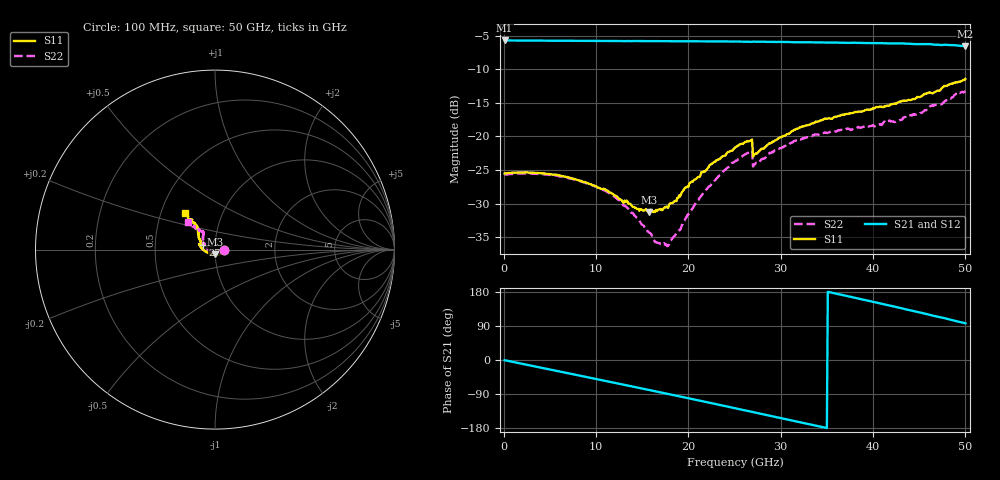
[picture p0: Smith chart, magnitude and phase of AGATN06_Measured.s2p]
! Filename4Jim: AG16_W2_AGATN06_B_0715_LRM_1BW_LRM.s2p
! Calibration: AG02 LRM + TRL
! Notes:
! Row:7, Col:15
! Probes: nan
! Prober: MPI TS150
! Date: 2023-09-21 10:47:37
! DC: None
# GHz S dB R 50
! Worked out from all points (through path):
!   500 points, 100 MHz to 50 GHz, reference 50 ohm
!   highest |S21| = -5.74 dB at 100 MHz (marker M1); lowest = -6.6 dB at 50 GHz (marker M2)
!   group delay of S21, straight-line fit = 14.5 ps
!   lowest |S11| = -31.3 dB at 15.7 GHz (marker M3), VSWR 1.06, Z = 50 - j2.71 ohm
!   |S11| at or under -10 dB: start of sweep to end of sweep
!   |S22| runs from -36.3 to -13.3 dB; largest |S21 - S12| = 0.00059
!   S11 on the Smith chart (normalised r, x): 100 MHz: 1.11, +0.00; 27 GHz: 0.88, +0.04; 50 GHz: 0.66, +0.29
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0.1  -25.54 0.1  -5.74 -0.5  -5.74 -0.5  -25.72 0.2
4.2  -25.52 -5.8  -5.77 -21.1  -5.77 -21.1  -25.64 -3.0
8.5  -26.72 -18.8  -5.79 -42.6  -5.79 -42.6  -26.77 -11.5
12.1  -28.87 -41.1  -5.81 -60.7  -5.81 -60.7  -29.09 -26.6
14.5  -30.82 -68.6  -5.82 -72.8  -5.82 -72.7  -32.23 -45.4
15.7  -31.33 -89.2  -5.82 -78.8  -5.82 -78.8  -34.27 -62.2
16.4  -31.26 -102.9  -5.83 -82.5  -5.83 -82.5  -35.72 -77.4
16.8  -30.90 -110.2  -5.83 -84.6  -5.83 -84.5  -35.90 -87.4
17.9  -30.22 -128.2  -5.85 -90.1  -5.85 -90.1  -36.04 -116.9
22  -24.96 -172.1  -5.88 -111.3  -5.88 -111.3  -27.86 176.0
25.1  -21.61 169.1  -5.89 -127.5  -5.89 -127.4  -23.64 157.5
26.7  -20.64 160.2  -5.93 -135.8  -5.93 -135.8  -22.26 150.8
27  -23.01 159.1  -5.91 -137.5  -5.91 -137.5  -24.49 154.4
27.2  -22.66 157.7  -5.91 -138.6  -5.91 -138.5  -24.16 153.4
29.5  -20.55 149.3  -5.94 -150.6  -5.95 -150.6  -22.03 143.4
33.4  -18.08 137.5  -6.02 -171.2  -6.02 -171.2  -19.97 131.2
37.7  -16.55 129.6  -6.07 165.9  -6.07 166.0  -19.01 125.2
41.7  -15.45 127.9  -6.18 144.1  -6.18 144.2  -17.72 126.0
45.1  -14.14 128.2  -6.28 125.1  -6.29 125.2  -16.53 129.7
46.2  -13.50 127.2  -6.28 118.7  -6.28 118.7  -15.46 132.6
49.1  -11.99 127.5  -6.49 102.0  -6.48 102.0  -13.55 133.4
50  -11.46 129.4  -6.58 97.0  -6.58 97.0  -13.31 133.7
